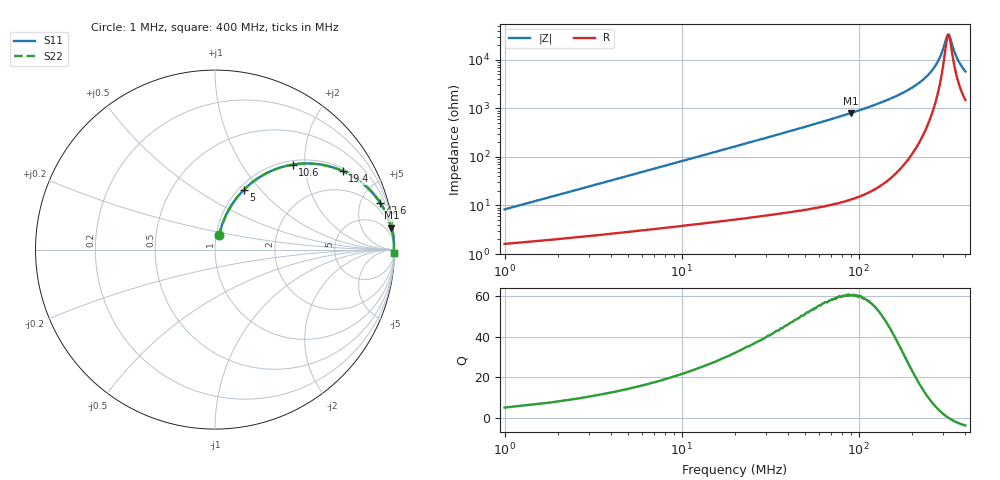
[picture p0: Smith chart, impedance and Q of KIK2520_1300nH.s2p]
!version-2
!date-01.2022
!Series
# MHz S RI R 50
!Freq ReS11 ImS11 ReS21 ImS21 ReS12 ImS12 ReS22 ImS22
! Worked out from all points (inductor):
!   500 points, 1 MHz to 400 MHz, reference 50 ohm
!   read as one part in series: L = 1.3 uH near 2.6 MHz
!   highest Q = 60.5 at 89.8 MHz (marker M1), where L = 1.41 uH
!   self-resonance near 321 MHz
!   S11 on the Smith chart (normalised r, x): 1 MHz: 1.03, +0.16; 5 MHz: 1.06, +0.82; 10.6 MHz: 1.08, +1.73; 19.4 MHz: 1.10, +3.18; 42.6 MHz: 1.15, +7.09; 400 MHz: open
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1  0.0222 0.0786  0.9778 -0.0786  0.9778 -0.0786  0.0222 0.0786
3.4  0.0908 0.2465  0.9092 -0.2465  0.9092 -0.2465  0.0908 0.2465
5  0.1602 0.3335  0.8398 -0.3335  0.8398 -0.3335  0.1602 0.3335
7.4  0.2792 0.4218  0.7208 -0.4218  0.7208 -0.4218  0.2792 0.4218
10.6  0.4325 0.4735  0.5675 -0.4735  0.5675 -0.4735  0.4325 0.4735
14.6  0.5854 0.4744  0.4146 -0.4744  0.4146 -0.4744  0.5854 0.4744
19.4  0.7108 0.4378  0.2892 -0.4378  0.2892 -0.4378  0.7108 0.4378
29  0.8446 0.3497  0.1554 -0.3497  0.1554 -0.3497  0.8446 0.3497
42.6  0.9216 0.2585  0.0784 -0.2585  0.0784 -0.2585  0.9216 0.2585
68.2  0.9688 0.1655  0.0312 -0.1655  0.0312 -0.1655  0.9688 0.1655
89.8  0.9825 0.1231  0.0175 -0.1231  0.0175 -0.1231  0.9825 0.1231
134  0.9929 0.0749  0.00713 -0.0749  0.00713 -0.0749  0.9929 0.0749
201  0.997 0.0368  0.00297 -0.0368  0.00297 -0.0368  0.997 0.0368
239  0.9975 0.0228  0.00245 -0.0228  0.00245 -0.0228  0.9975 0.0228
267  0.9976 0.0141  0.00244 -0.0141  0.00244 -0.0141  0.9976 0.0141
291  0.9974 0.00754  0.00261 -0.00754  0.00261 -0.00754  0.9974 0.00754
316  0.9971 0.00115  0.00293 -0.00115  0.00293 -0.00115  0.9971 0.00115
323  0.997 -0.00036  0.00303 0.00036  0.00303 0.00036  0.997 -0.00036
334  0.9968 -0.00293  0.00322 0.00293  0.00322 0.00293  0.9968 -0.00293
344  0.9966 -0.00524  0.00342 0.00524  0.00342 0.00524  0.9966 -0.00524
360  0.9963 -0.00867  0.00375 0.00867  0.00375 0.00867  0.9963 -0.00867
400  0.9953 -0.0166  0.00471 0.0166  0.00471 0.0166  0.9953 -0.0166
